FUNCTION_BLOCK FB21
TITLE =Get Current Must
//*****************************************************************************
//* maxon motor ag
//* R&D
//* all rights reserved
//*****************************************************************************
//* Summary:  Read demand value of current
//*
//* Remarks:
//*
//* Created under: STEP7 REV5.2+SP1
//*****************************************************************************
//* History:
//* 19.05.2004 | INA   first release
//*
//*
//*****************************************************************************
//

AUTHOR:INA
FAMILY:CurrentM
NAME:GetCurM
VERSION:00.01


VAR_INPUT

Read : BOOL //A rising edge start the command

  NodeID : BYTE //Adress of the maxon device

END_VAR
VAR_OUTPUT
  Done : BOOL //Data valid flag is TRUE if data were available

  Err : BOOL //Error flag is TRUE if an Error has occured, see ErrNo for more details

  ErrNo : DINT //Contains detailed error information

  CurrentMust : WORD //Current mode demand value

END_VAR
VAR
  xEdgeMerker : BOOL //Edge Merker

  xEdgeFlag : BOOL //Edge Flag

  xStep : INT
END_VAR

BEGIN

NETWORK
TITLE = Activate the service function
//

// SDO Read "Get Current Must"

       U    #Read
       FP   #xEdgeFlag                   // recognize a positiv edge of the Read signal
       =    #xEdgeMerker                 // and set the xEdgeMerker for one cycle to true

       L    #xStep
       L    0
       ==I
       U    #xEdgeMerker
       SPB  nstp                         // iStep = 1 -> fnc1

       L    #xStep                       // jump list
       SPL  List
       SPA  rdef
       SPA  fnc1
       SPA  fncE
List  :SPA  rdef

rdef  :NOP  0
       R    #Done                        // reset Done
       R    #Err                         // reset Error
       L    0
       T    #xStep                       // iStep = 0
       SPA  end

fnc1  :NOP  0

       CALL FC1
         NodeID:=#NodeID
         Index:=DW#16#00002030
         SubIndex:=DW#16#00000000
         RET_VAL:=#Done
         Err:=#Err
         ErrNo:=#ErrNo

       L    DB219.DBW10
       T    #CurrentMust

fncE  :NOP  0
       L    0
       T    #xStep
       SPA  end

nstp  :NOP  0
       L    #xStep
       INC            1
       T    #xStep

end   :NOP  0
END_FUNCTION_BLOCK
